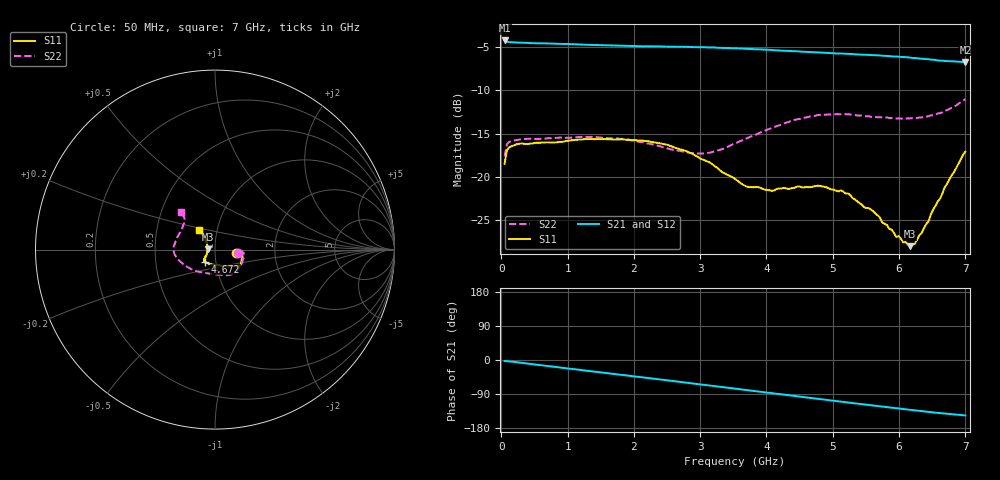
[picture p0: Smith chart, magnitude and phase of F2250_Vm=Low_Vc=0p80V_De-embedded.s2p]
! Integrated Device Technology
! Corporate Headquarters
! 6024 Silver Creek Valley Road
! San Jose, CA 95138  USA
! Phone:  1-408-284-8200
! Toll Free:  1-800-223-1366
! Webpage:  http://www.idt.com/
! Timing and RF Division
! 515 Groton Road, Suite 102
! Westford, MA 01886-6024
! Device:  F2250
! Description: Voltage Variable RF Attenuator
! Frequency:  50.0 -  6000.00 MHz
! Package:  3x3 mm Thin QFN Plastic Package: 16 pin
! Ports:  2 RF, 3 DC
!  Pin  1  = GND
!  Pin  2  = NC
!  Pin  3  = RF1  = Port 1
!  Pin  4  = NC
!  Pin  5  = GND
!  Pin  6  = GND
!  Pin  7  = GND
!  Pin  8  = GND
!  Pin  9  = NC
!  Pin 10  = RF2  = Port 2
!  Pin 11  = NC
!  Pin 12  = GND
!  Pin 13  = GND
!  Pin 14  = VCNTRL
!  Pin 15  = VDD
!  Pin 16  = VMODE
! Vcntrl:  0.800 Volts
! Vmode:  +0.000 Volts
! Vdd:  +3.30  Volts
! Current:  1.165 mA
! Data:  The device was measured on a the F2250 evaluation board which has
!  individual transmission lines to the RF pins.  Data was collected
!  using a calibrated network analyzer.  The evaluation board was
!  de-embedded using a TRL calibration technique.
!  The reference plane is the edge of the package pin.
! Misc:  SN 10
!  Action Tracker AT0258
! Date Measured:  2014-11-26
! Date:  2015-10-15  MJV
! Note:
!  Integrated Device Technology supplies this data as a sample of measured
!  data at the package pin for this product.  Your particular data for this
!  product may vary.
!  Data was taken at 25 degrees C.
!  Integrated Device Technology reserves the right to change this data at anytime.
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# GHz S dB R 50
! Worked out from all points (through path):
!   201 points, 50 MHz to 7 GHz, reference 50 ohm
!   highest |S21| = -4.21 dB at 50 MHz (marker M1); lowest = -6.7 dB at 7 GHz (marker M2)
!   group delay of S21, straight-line fit = 58.7 ps
!   lowest |S11| = -28.0 dB at 6.166 GHz (marker M3), VSWR 1.08, Z = 46.2 + j0.208 ohm
!   |S11| at or under -10 dB: start of sweep to end of sweep
!   |S22| runs from -17.6 to -11.0 dB; largest |S21 - S12| = 0.0012
!   S11 on the Smith chart (normalised r, x): 50 MHz: 1.27, -0.04; 4.672 GHz: 0.89, -0.12; 7 GHz: 0.82, +0.18
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0.05  -18.47 -7.8  -4.21 -2.8  -4.22 -2.8  -17.64 -8.2
0.08475  -16.90 -5.2  -4.35 -3.1  -4.36 -3.1  -16.22 -6.0
0.22375  -16.24 -6.9  -4.44 -5.7  -4.45 -5.7  -15.74 -9.6
1.2315  -15.66 -28.3  -4.70 -27.2  -4.71 -27.2  -15.37 -43.4
1.857  -15.69 -33.7  -4.83 -40.1  -4.83 -40.1  -15.62 -57.8
2.37825  -16.08 -36.2  -4.90 -51.0  -4.91 -51.0  -16.42 -70.4
2.79525  -17.02 -41.0  -4.95 -59.9  -4.96 -59.9  -17.15 -87.2
3.0385  -18.00 -46.6  -5.00 -65.2  -4.99 -65.2  -17.30 -100.6
3.525  -20.22 -67.5  -5.11 -75.8  -5.12 -75.8  -16.13 -128.7
3.69875  -21.11 -78.6  -5.18 -79.6  -5.19 -79.6  -15.54 -137.3
4.081  -21.61 -103.5  -5.32 -87.9  -5.33 -87.9  -14.34 -154.1
4.67175  -21.19 -129.4  -5.57 -100.6  -5.56 -100.6  -12.97 -171.8
4.7065  -21.11 -130.5  -5.57 -101.3  -5.56 -101.3  -12.96 -172.6
5.22775  -21.91 -139.3  -5.77 -112.2  -5.77 -112.2  -12.76 175.7
5.471  -23.50 -142.2  -5.87 -117.2  -5.88 -117.2  -12.98 170.0
5.61  -23.97 -144.1  -5.90 -120.1  -5.91 -120.1  -13.09 166.3
5.85325  -26.02 -153.7  -6.02 -125.1  -6.03 -125.1  -13.19 159.9
6.166  -28.01 176.8  -6.19 -131.5  -6.21 -131.5  -13.23 150.2
6.2355  -27.74 164.8  -6.24 -132.9  -6.24 -133.0  -13.21 147.6
6.444  -25.14 142.6  -6.38 -137.1  -6.39 -137.1  -12.99 141.0
6.68725  -21.20 130.5  -6.59 -141.3  -6.59 -141.3  -12.34 134.6
7  -17.08 130.2  -6.71 -146.3  -6.71 -146.4  -11.01 132.1
